| IBIS file generated by GenIBIS323.exe Version 3.23
|   TDA2x
[IBIS ver]   5.0
[File name]   TDA2x.ibs
[File Rev]   1.3.4
[Date]   Mon Apr 15, 2014, 10:23:51
[Source]   Data created at Texas Instruments
[Notes]   TDA2x 23mm IBIS Model Revision History
   TDA2x Version 1.3.4, June 9th, 2014
   - Created TDA2x version from parent device
   - Does not apply to TDA2Ex device
   Version 1.3.4, April 15, 2014
   - Added new 1-2-1 package RLC data
   Version 1.3.3, September 20, 2013
   - Updated the following models to more accurately
   represent the slew and delay characteristics.
   * Models include:
   > bc1833dv40dcpbfbhhvrxp1811_sscev
   > bc1833dv40dcpbfbp1811_ssceh
   > bc1833dv40dcpbfbp1811_sscev
   > bi2c1833dvfzp18_sscev
   > iq1833dvtckpbfbp18ll_sscev
   * Peripherals that use the corresponding IO buffers
   include:
   > GPMC
   > VIN/VOUT
   > MDIO
   > RGMII
   > UART
   > McASP
   > GPIO
   > MMC
   > SPI
   > DCAN
   > I2C
   > USB (AB10,AC10)
   > Debug
   > System and Misc Signals
   Version 1.3.2, August 14, 2013
   - Updated DDR models to address the minimum supply
   voltage and the discontinuities in the vertical
   single ended models.
   Version 1.3.1, August 5, 2013
   - Updated DDR2 (1.8V) models; regenerated at 400 MHz
   Version 1.3.0, June 14, 2013
   - Added I2C models
   - Added MLB models
   - Added DDR Clock pins as differential
   Version 1.2.0, May 23, 2013
   - Added DDR2 (1.8V) models
   - Added DDR DQS pins as differential
   Version 1.1.1, April 8, 2013
   - Modifications, Additions, Deletions
   * Changed name of file to be package specific
   * Updated the following source IO models:
   > DDR_SEIOPB_V
   > DDR_SEIOPB_H
   > DDR_DIFFIOPB_H
   * Replaced the following source IO models:
   > GANGARX_HMAV10GS80 with GANGARX
   > SHANTANUTX_HMAV10GS80 with
   USB3_PCIEGEN1_PCIEGEN2_TX / SATATX
   * Added the following source IO models:
   > ACSPCIE_RX
   > IHHV1833DVHYP1811_SSCEV
   > BC1833DV40DCPBFBHHVRXP1811_SSCEV
   > IQ1833DVTCKPBFBP18LL_SSCEV
   * Changed source IO buffer model to existing model
   > For some pins, the following two models were
   interchanged: BC1833DV40DCPBFBP1811_SSCEH,
   BC1833DV40DCPBFBP1811_SSCEV
   * Updated the RLC data for all pins
   * Changed the supported DDR voltage from 1.2V/1.5V
   to 1.35/1.5V for DDR3 usage
   Version 1.0, January 16, 2013
   - Initial Release
   Note 1) Checked by IBISCHK5.
   Note 2) Interfaces Included in this IBIS Model
   - DDR1,2
   - GPIO6
   - GPMC
   - VIP1
   - VIP2
   - DSS
   - HDMI1
   - RGMII
   - UART3
   - USB1,2
   - PCIE
   - XREFCLK
   - McASP1,2,3,4,5
   - MMC1,3
   - SPI1,2
   - DCAN
   - UART1,2,3
   - SATA1
   - I2C1
   - I2C2
   - MLB
[Disclaimer] Please be aware that in the absence of a written agreement,
   Texas Instruments (TI) assumes no liability for: 1) the
   accuracy of the IBIS models provided to your company, 2) the
   proper functioning of these IBIS models in your design or for
   any resulting applications, or, 3) infringement of patents,
   copyrights, or intellectual property rights resulting from
   your use of these IBIS models. TI provides IBIS models as a
   service to our customers and therefore reserves the right to
   limit distribution of the IBIS models.
[Copyright]   Property of Texas Instruments Incorporated. Unauthorised
   reproduction and/or distribution is strictly prohibited. This
   product is protected under copyright law and trade secret law
   as an unpublished work. Created 2013,(C) Copyright 2013,
   Texas Instruments Incorporated., All Rights Reserved. These
   commodities are under the U.S. Government distribution license
   control.As such,they are not to be re-exported without the
   prior approval of the U.S. Department of Commerce.
|   Component TDA2x
[Component]   TDA2x
[Manufacturer]   Texas Instruments.
| Source IO level model revisions
|Model   Revision   Date
|ILVDS18HY_SSCEH   1.0   Apr 04, 2013
|BMLBLVDS18_SSCEH   1.0   Jun 13, 2013
|BC1833DV40DCPBFBP1811_SSCEH   2.0   Sep 11, 2013
|DDR_SEIOPB_H   2.4   14 Aug 2013
|GANGARX   1   Sep 04, 2012
|SDIO1833PB_H   1.0   Sep 21, 2011
|IQ1833DVTCKPBFBP18LL_SSCEV   2.0   Sep 11, 2013
|USB3_PCIEGEN1_PCIEGEN2_TX   1.0   Nov 07, 2012
|ACSPCIE_RX   0.5   May 16, 2012
|BI2C1833DVFZP18_SSCEV   2.0   Sep 11, 2013
|IHHV1833DVHYP1811_SSCEV   1.0   Dec 24, 2012
|DDR_SEIOPB_V   2.4   14 Aug 2013
|DDR_DIFFIOPB_H   2.4   14 Aug 2013
|HDMITXPHY   0.8   Jul 12, 2011
|DDR_DIFFIOPB_V   2.4   14 Aug 2013
|USB2PHYCORE_HMAV10GS80   0.8   July 13, 2011
|BC1833DV40DCPBFBP1811_SSCEV   2.0   Sep 11, 2013
|SATATX   1.0   Nov 07, 2012
|BC1833DV40DCPBFBHHVRXP1811_SSCEV   2.0   Sep 11, 2013
[Package]
|   typ   min   max
R_pkg   0.410630813888888   0.0487026   0.806879
L_pkg   5.77142293162393E-009 8.65672E-10   1.23044E-08
C_pkg   7.4889892948718E-013 2.85269E-13   1.26574E-12
[Pin]   signal_name   model_name   R_pin   L_pin   C_pin
Y10   ATESTV   NC
G19   DCAN1_RX   Selector_10  0.142301   1.81835E-09 4.38728E-13
G20   DCAN1_TX   Selector_10  0.137913   1.91785E-09 4.43391E-13
AA25   DDR1_D30   Selector_9   0.488374   6.55624E-09 9.83881E-13
AC26   DDR1_DQM2   Selector_23  0.571621   7.36463E-09 7.5871E-13
AA27   DDR1_DQM3   Selector_23  0.505641   7.39922E-09 8.05209E-13
AH22   DDR1_A5   Selector_14  0.489767   6.96396E-09 8.56083E-13
Y27   DDR1_DQSN3   Selector_22  0.468375   7.13463E-09 6.18565E-13
AA26   DDR1_D29   Selector_9   0.504051   6.68279E-09 8.96047E-13
Y20   DDR1_D23   Selector_9   0.455055   4.62626E-09 9.31601E-13
AF25   DDR1_D0   Selector_9   0.547194   7.82073E-09 8.17645E-13
AD27   DDR1_DQS2   Selector_2   0.511052   7.93612E-09 6.63607E-13
V20   DDR1_D16   Selector_9   0.496658   4.60207E-09 6.66551E-13
AE28   DDR1_DQSN1   Selector_22  0.52608   8.75962E-09 6.7652E-13
W22   DDR1_ECC_D0   Selector_9   0.391173   4.73415E-09 8.7308E-13
W20   DDR1_D17   Selector_9   0.476985   4.28121E-09 8.48532E-13
Y23   DDR1_D26   Selector_9   0.479951   5.39702E-09 8.38804E-13
AD20   DDR1_A0   Selector_14  0.491074   4.69941E-09 7.61683E-13
AD22   DDR1_A11   Selector_14  0.464556   5.06886E-09 7.34666E-13
AD18   DDR1_A15   Selector_14  0.477384   4.97278E-09 7.25895E-13
AH25   DDR1_DQS0   Selector_2   0.491307   7.94468E-09 6.51776E-13
AF28   DDR1_D11   Selector_9   0.563042   8.80825E-09 9.29844E-13
AH21   DDR1_WEN   Selector_14  0.490909   6.72126E-09 7.52517E-13
AC18   DDR1_CASN   Selector_14  0.479809   4.10908E-09 9.02863E-13
Y25   DDR1_ECC_D4   Selector_9   0.433519   6.03553E-09 8.75322E-13
AF23   DDR1_D6   Selector_9   0.525055   6.82231E-09 9.6887E-13
AC19   DDR1_A1   Selector_14  0.465932   4.58919E-09 8.99261E-13
AE24   DDR1_D5   Selector_9   0.567056   6.70164E-09 8.95563E-13
AF21   DDR1_A4   Selector_14  0.465648   5.66338E-09 8.01622E-13
AE21   DDR1_A7   Selector_14  0.4759   5.50088E-09 7.72657E-13
AC27   DDR1_D20   Selector_9   0.548177   7.71401E-09 9.67757E-13
AA24   DDR1_D27   Selector_9   0.485891   5.99486E-09 1.02065E-12
V28   DDR1_DQSN_ECC   Selector_22  0.428445   6.8489E-09 5.83984E-13
AH23   DDR1_CSN0   Selector_14  0.485959   7.33449E-09 8.46496E-13
V25   DDR1_ECC_D6   Selector_9   0.442687   5.42329E-09 8.91358E-13
AE26   DDR1_D12   Selector_9   0.564674   7.86732E-09 1.01558E-12
W19   DDR1_ECC_D2   Selector_9   0.305263   4.60654E-09 4.91779E-13
AF27   DDR1_D9   Selector_9   0.565294   8.17506E-09 1.03913E-12
V24   DDR1_ECC_D5   Selector_9   0.433492   5.15658E-09 1.03737E-12
AD23   DDR1_DQM0   Selector_23  0.535358   5.90176E-09 7.25313E-13
AC21   DDR1_A12   Selector_14  0.444582   4.2461E-09 6.71249E-13
Y18   DDR1_VREF0   NC
AF22   DDR1_A8   Selector_14  0.482908   5.98594E-09 8.51919E-13
V23   DDR1_ECC_D1   Selector_9   0.410952   4.86996E-09 8.7205E-13
Y28   DDR1_DQS3   Selector_2   0.469432   7.46481E-09 6.15791E-13
AF20   DDR1_RASN   Selector_14  0.492836   6.17494E-09 7.29374E-13
AG24   DDR1_CK   Selector_7   0.463144   7.46419E-09 6.60615E-13
AD28   DDR1_DQSN2   Selector_22  0.510404   8.32224E-09 6.74162E-13
AB18   DDR1_BA2   Selector_14  0.476485   3.73249E-09 7.57707E-13
AC25   DDR1_D13   Selector_9   0.561034   6.53819E-09 9.74056E-13
AH26   DDR1_D3   Selector_9   0.563544   8.67391E-09 9.23805E-13
AG23   DDR1_A6   Selector_14  0.477168   6.94389E-09 7.82961E-13
AF24   DDR1_D4   Selector_9   0.567364   7.24396E-09 9.65163E-13
AA28   DDR1_D31   Selector_9   0.505301   7.57104E-09 8.85626E-13
AB19   DDR1_A3   Selector_14  0.458874   3.63375E-09 7.35145E-13
Y24   DDR1_D28   Selector_9   0.486596   5.86172E-09 1.08233E-12
V27   DDR1_DQS_ECC   Selector_2   0.422662   6.40168E-09 6.29942E-13
AA23   DDR1_D24   Selector_9   0.460929   6.1893E-09 9.79318E-13
AF18   DDR1_A13   Selector_14  0.429673   5.58028E-09 7.25804E-13
AC23   DDR1_D8   Selector_9   0.538858   6.26131E-09 7.73819E-13
AC28   DDR1_D19   Selector_9   0.544104   8.03812E-09 9.71096E-13
AE23   DDR1_D7   Selector_9   0.543229   6.3764E-09 9.88105E-13
AE18   DDR1_BA1   Selector_14  0.448614   5.33588E-09 8.03247E-13
AB23   DDR1_DQM1   Selector_23  0.53767   6.04637E-09 9.46043E-13
Y19   DDR1_D21   Selector_9   0.448452   4.88152E-09 9.80373E-13
AG26   DDR1_D2   Selector_9   0.566242   8.35538E-09 9.98633E-13
AH24   DDR1_NCK   Selector_18  0.463978   7.70005E-09 6.37576E-13
V26   DDR1_DQM_ECC   Selector_23  0.461108   6.09944E-09 7.12956E-13
AE17   DDR1_A14   Selector_14  0.393257   4.55887E-09 6.9875E-13
AG25   DDR1_DQSN0   Selector_22  0.488286   7.6544E-09 6.85193E-13
AE20   DDR1_ODT0   Selector_14  0.493335   5.59178E-09 8.74184E-13
Y22   DDR1_D25   Selector_9   0.455152   5.4378E-09 8.79622E-13
AC24   DDR1_D14   Selector_9   0.562772   6.40383E-09 9.77754E-13
AC20   DDR1_A2   Selector_14  0.474437   4.33433E-09 8.21491E-13
AE22   DDR1_A9   Selector_14  0.451572   5.54208E-09 7.5977E-13
AD25   DDR1_D15   Selector_9   0.563905   7.18622E-09 8.33158E-13
AB27   DDR1_D22   Selector_9   0.548017   7.16469E-09 9.34631E-13
AF17   DDR1_BA0   Selector_14  0.363148   5.09595E-09 7.8349E-13
W23   DDR1_ECC_D3   Selector_9   0.411229   5.50469E-09 8.04349E-13
AB28   DDR1_D18   Selector_9   0.548364   7.9815E-09 8.83095E-13
AF26   DDR1_D1   Selector_9   0.564992   7.96636E-09 8.38444E-13
Y26   DDR1_ECC_D7   Selector_9   0.437804   6.33869E-09 8.243E-13
AG22   DDR1_CKE   Selector_14  0.488524   6.8453E-09 8.89617E-13
AE27   DDR1_DQS1   Selector_2   0.527341   8.41091E-09 7.07295E-13
AD21   DDR1_A10   Selector_14  0.450742   4.90139E-09 7.69093E-13
AG21   DDR1_RST   Selector_14  0.465812   6.64602E-09 6.81961E-13
AG27   DDR1_D10   Selector_9   0.563089   8.64448E-09 9.80341E-13
P25   DDR2_A6   Selector_23  0.453003   5.94758E-09 9.09075E-13
G28   DDR2_DQS0   Selector_2   0.461291   7.57794E-09 6.16914E-13
T23   DDR2_RASN   Selector_23  0.412552   5.07283E-09 9.11349E-13
M25   DDR2_D30   Selector_9   0.429649   4.93162E-09 8.66061E-13
M24   DDR2_D29   Selector_9   0.425194   4.32737E-09 8.16752E-13
R27   DDR2_A3   Selector_23  0.474573   6.03892E-09 8.14153E-13
R25   DDR2_A0   Selector_23  0.480037   5.494E-09  1.03762E-12
H28   DDR2_DQSN1   Selector_22  0.416577   6.83933E-09 5.59439E-13
J24   DDR2_D15   Selector_9   0.445443   4.53076E-09 7.05822E-13
G24   DDR2_DQM1   Selector_23  0.413019   5.05315E-09 9.52893E-13
P27   DDR2_A8   Selector_23  0.478091   6.65855E-09 7.30202E-13
L25   DDR2_D26   Selector_9   0.419384   4.9549E-09 6.50443E-13
F26   DDR2_D4   Selector_9   0.478471   5.90808E-09 8.82784E-13
N23   DDR2_A10   Selector_23  0.424246   5.70493E-09 8.87666E-13
P23   DDR2_A4   Selector_23  0.435404   5.35545E-09 1.03205E-12
H27   DDR2_DQS1   Selector_2   0.41834   6.40587E-09 5.8892E-13
U23   DDR2_BA0   Selector_23  0.429682   5.52565E-09 9.25158E-13
H25   DDR2_D9   Selector_9   0.444286   4.73335E-09 7.78562E-13
K28   DDR2_DQSN2   Selector_22  0.388299   6.17591E-09 5.59537E-13
T22   DDR2_A13   Selector_23  0.435755   4.62863E-09 8.39607E-13
U24   DDR2_CKE   Selector_23  0.417375   6.15441E-09 1.08206E-12
E28   DDR2_D7   Selector_9   0.420185   6.68015E-09 9.52895E-13
J26   DDR2_D14   Selector_9   0.444455   5.43806E-09 8.14335E-13
K22   DDR2_D22   Selector_9   0.407858   3.17351E-09 7.19244E-13
F27   DDR2_D5   Selector_9   0.47131   6.27857E-09 8.77333E-13
N22   DDR2_VREF0   NC
R24   DDR2_RST   Selector_23  0.459467   4.75459E-09 6.10277E-13
N27   DDR2_A9   Selector_23  0.500555   6.42607E-09 8.0858E-13
H24   DDR2_D10   Selector_9   0.444695   4.26735E-09 6.84693E-13
E26   DDR2_D0   Selector_9   0.430381   6.16167E-09 9.3642E-13
G27   DDR2_DQSN0   Selector_22  0.458967   7.12203E-09 6.88688E-13
L26   DDR2_D25   Selector_9   0.434294   5.28274E-09 7.6646E-13
R23   DDR2_ODT0   Selector_23  0.454898   4.84341E-09 9.81403E-13
L23   DDR2_D19   Selector_9   0.405574   3.83659E-09 6.59391E-13
N28   DDR2_A12   Selector_23  0.486579   6.7043E-09 6.97861E-13
H23   DDR2_D8   Selector_9   0.450297   3.89798E-09 5.15707E-13
P26   DDR2_A11   Selector_23  0.27554   5.36883E-09 8.32604E-13
M22   DDR2_DQM3   Selector_23  0.433598   3.74065E-09 6.35021E-13
P24   DDR2_CSN0   Selector_23  0.443812   5.65757E-09 1.04452E-12
U25   DDR2_WEN   Selector_23  0.465624   5.85963E-09 8.43561E-13
K21   DDR2_D18   Selector_9   0.379168   3.3037E-09 6.88322E-13
K23   DDR2_DQM2   Selector_23  0.406601   3.77847E-09 6.3791E-13
J25   DDR2_D13   Selector_9   0.444619   4.87823E-09 7.98274E-13
M23   DDR2_D28   Selector_9   0.427683   3.80719E-09 6.64654E-13
G26   DDR2_D12   Selector_9   0.443789   5.60773E-09 8.27383E-13
U26   DDR2_BA2   Selector_23  0.479623   5.80667E-09 9.01941E-13
L27   DDR2_D24   Selector_9   0.434949   6.03771E-09 8.29766E-13
M27   DDR2_DQSN3   Selector_22  0.404049   6.195E-09  5.77957E-13
P22   DDR2_A5   Selector_23  0.429797   5.34435E-09 9.09059E-13
J23   DDR2_D21   Selector_9   0.35896   4.27659E-09 7.56671E-13
E27   DDR2_D6   Selector_9   0.424828   6.27032E-09 8.80003E-13
M26   DDR2_D31   Selector_9   0.428812   5.21643E-09 7.91056E-13
K20   DDR2_D17   Selector_9   0.363681   2.97052E-09 7.84333E-13
R28   DDR2_A2   Selector_23  0.440338   6.66525E-09 8.68351E-13
M28   DDR2_DQS3   Selector_2   0.403534   6.65019E-09 5.74802E-13
F25   DDR2_D2   Selector_9   0.475806   5.54542E-09 9.76788E-13
L24   DDR2_D20   Selector_9   0.405479   4.09588E-09 6.63414E-13
F28   DDR2_DQM0   Selector_23  0.496294   7.81995E-09 5.88209E-13
H26   DDR2_D11   Selector_9   0.445756   5.128E-09  8.01138E-13
K27   DDR2_DQS2   Selector_2   0.389027   5.94231E-09 5.4361E-13
R22   DDR2_A14   Selector_23  0.431613   4.10396E-09 7.31404E-13
G25   DDR2_D1   Selector_9   0.491438   5.25161E-09 6.80725E-13
U28   DDR2_CASN   Selector_23  0.479485   6.88158E-09 8.56654E-13
L28   DDR2_D27   Selector_9   0.431477   6.08946E-09 7.63716E-13
T27   DDR2_NCK   Selector_19  0.451957   6.99093E-09 6.55098E-13
U27   DDR2_BA1   Selector_23  0.48795   6.26323E-09 8.69074E-13
R26   DDR2_A1   Selector_23  0.445263   5.56403E-09 1.06848E-12
J20   DDR2_D23   Selector_9   0.351626   3.25197E-09 7.55244E-13
F24   DDR2_D3   Selector_9   0.475631   5.2045E-09 8.98858E-13
T28   DDR2_CK   Selector_20  0.45108   7.27277E-09 6.2314E-13
L22   DDR2_D16   Selector_9   0.402625   3.21383E-09 6.02036E-13
N20   DDR2_A7   Selector_23  0.432107   3.79928E-09 8.42539E-13
U22   DDR2_A15   Selector_23  0.407669   5.35849E-09 8.89981E-13
G21   EMU0   Selector_10  0.183887   2.70625E-09 5.53086E-13
D24   EMU1   Selector_10  0.571856   8.40046E-09 1.04504E-12
F21   GPIO6_16   Selector_10  0.225689   3.20669E-09 5.5591E-13
E21   GPIO6_14   Selector_10  0.303084   4.38462E-09 5.03666E-13
AC5   GPIO6_10   Selector_5   0.474075   6.7728E-09 8.64123E-13
AB4   GPIO6_11   Selector_5   0.421245   6.01837E-09 7.04268E-13
F20   GPIO6_15   Selector_10  0.212065   2.77626E-09 4.91169E-13
P3   GPMC_A17   Selector_5   0.371938   5.45505E-09 7.36827E-13
R6   GPMC_A0   Selector_5   0.217732   2.94649E-09 5.55936E-13
J4   GPMC_A24   Selector_5   0.247695   3.62428E-09 5.05395E-13
J3   GPMC_AD13   Selector_5   0.315242   4.72363E-09 6.92293E-13
L1   GPMC_AD8   Selector_5   0.449743   6.93734E-09 7.28573E-13
P5   GPMC_A7   Selector_5   0.246699   3.17065E-09 5.81908E-13
P6   GPMC_A4   Selector_5   0.17379   2.40117E-09 5.00132E-13
P1   GPMC_CS3   Selector_5   0.486377   7.23655E-09 7.86426E-13
M7   GPMC_A20   Selector_5   0.237756   4.28796E-09 8.09544E-13
L5   GPMC_AD2   Selector_5   0.21652   3.006E-09  5.05478E-13
R3   GPMC_A13   Selector_5   0.417385   5.8408E-09 8.1052E-13
L4   GPMC_AD5   Selector_5   0.237065   3.57808E-09 5.1762E-13
H5   GPMC_A27   Selector_5   0.220691   3.08692E-09 4.66919E-13
P4   GPMC_A12   Selector_5   0.270486   3.84668E-09 6.33659E-13
J1   GPMC_AD10   Selector_5   0.461393   6.84793E-09 7.51707E-13
M1   GPMC_AD3   Selector_5   0.431467   6.64752E-09 6.5277E-13
T9   GPMC_A1   Selector_5   0.297577   4.20392E-09 7.47103E-13
H2   GPMC_AD14   Selector_5   0.424887   6.22548E-09 7.87734E-13
M6   GPMC_AD0   Selector_5   0.0623967  1.73897E-09 4.65864E-13
N6   GPMC_BEN0   Selector_5   0.181144   2.4119E-09 5.23354E-13
M2   GPMC_AD1   Selector_5   0.36614   5.551E-09  6.95395E-13
R2   GPMC_A18   Selector_5   0.426261   6.45202E-09 8.30275E-13
J6   GPMC_A25   Selector_5   0.161418   2.31366E-09 4.44825E-13
R4   GPMC_A9   Selector_5   0.364075   4.69363E-09 6.6057E-13
N9   GPMC_A10   Selector_5   0.0704516  1.39445E-09 3.71414E-13
L6   GPMC_AD4   Selector_5   0.0628788  1.65793E-09 4.75715E-13
R5   GPMC_A6   Selector_5   0.314166   4.15121E-09 6.70616E-13
M4   GPMC_BEN1   Selector_5   0.284796   3.91097E-09 5.91591E-13
H1   GPMC_AD12   Selector_5   0.49008   7.25447E-09 7.7463E-13
T6   GPMC_A2   Selector_5   0.310609   4.31386E-09 6.68677E-13
J2   GPMC_AD11   Selector_5   0.37862   5.63845E-09 7.86007E-13
T1   GPMC_CS0   Selector_5   0.547747   8.08251E-09 8.63303E-13
H6   GPMC_CS1   Selector_5   0.15283   2.16164E-09 3.54794E-13
H3   GPMC_AD15   Selector_5   0.366945   5.27839E-09 6.29529E-13
T2   GPMC_A14   Selector_5   0.45378   6.55015E-09 8.93429E-13
U2   GPMC_A15   Selector_5   0.539544   7.78702E-09 9.79267E-13
N1   GPMC_ADVN_ALE   Selector_5   0.473783   6.96964E-09 7.42842E-13
N2   GPMC_WAIT0   Selector_5   0.382117   5.7663E-09 7.56475E-13
J5   GPMC_A21   Selector_5   0.188381   2.77218E-09 4.57131E-13
P7   GPMC_CLK   Selector_5   0.0817759  1.29823E-09 4.9009E-13
R9   GPMC_A5   Selector_5   0.251842   3.75325E-09 6.67436E-13
K7   GPMC_A19   Selector_5   0.111553   1.59599E-09 4.21047E-13
U1   GPMC_A16   Selector_5   0.539046   7.94879E-09 8.44175E-13
N7   GPMC_A8   Selector_5   0.182345   2.10979E-09 5.97325E-13
M3   GPMC_WEN   Selector_5   0.345682   4.91728E-09 6.73703E-13
J7   GPMC_A23   Selector_5   0.10285   1.48507E-09 3.77069E-13
T7   GPMC_A3   Selector_5   0.212634   3.28461E-09 7.98296E-13
P2   GPMC_CS2   Selector_5   0.397616   5.96876E-09 7.88128E-13
M5   GPMC_OEN_REN   Selector_5   0.199781   2.88885E-09 5.41255E-13
P9   GPMC_A11   Selector_5   0.120642   2.00577E-09 5.14429E-13
L2   GPMC_AD7   Selector_5   0.359214   5.58E-09   6.93076E-13
L3   GPMC_AD6   Selector_5   0.325981   4.87955E-09 6.17128E-13
H4   GPMC_A26   Selector_5   0.252297   3.65141E-09 5.21147E-13
K2   GPMC_AD9   Selector_5   0.351971   5.59305E-09 6.4468E-13
K6   GPMC_A22   Selector_5   0.200506   2.50226E-09 4.82556E-13
AH16   HDMI1_CLOCKY   Model_560   0.522079   6.86158E-09 5.59959E-13
AH17   HDMI1_DATA0Y   Model_560   0.54149   6.98311E-09 5.71255E-13
AH19   HDMI1_DATA2Y   Model_560   0.540501   7.19948E-09 5.3239E-13
AG16   HDMI1_CLOCKX   Model_559   0.519718   6.47654E-09 5.30151E-13
AH18   HDMI1_DATA1Y   Model_560   0.526848   7.01394E-09 5.91894E-13
AG18   HDMI1_DATA1X   Model_559   0.513665   6.3596E-09 6.08132E-13
AG19   HDMI1_DATA2X   Model_559   0.540457   6.6137E-09 5.66E-13
AG17   HDMI1_DATA0X   Model_559   0.537899   6.51607E-09 5.86014E-13
C20   I2C1_SCL   Selector_4   0.391047   5.4679E-09 7.3579E-13
F17   I2C2_SCL   Selector_4   0.158122   2.18035E-09 5.01077E-13
C21   I2C1_SDA   Selector_4   0.395798   5.82709E-09 8.22531E-13
C25   I2C2_SDA   Selector_4   0.64304   9.74271E-09 8.75737E-13
AH15   LJCB_CLKN   Model_228   0.403117   6.62067E-09 5.54035E-13
AG15   LJCB_CLKP   Model_228   0.402119   6.35043E-09 5.88998E-13
E12   MCASP1_AXR4   Selector_10  0.228305   3.05529E-09 5.26292E-13
B14   MCASP1_ACLKR   Selector_10  0.333237   4.81969E-09 7.15725E-13
G13   MCASP1_AXR2   Selector_10  0.114295   1.47199E-09 4.72026E-13
A11   MCASP1_AXR9   Selector_10  0.464424   7.04465E-09 6.57801E-13
G12   MCASP1_AXR0   Selector_10  0.073142   1.12741E-09 4.05063E-13
D14   MCASP1_FSX   Selector_10  0.211293   3.11931E-09 5.35981E-13
G14   MCASP1_AXR14   Selector_10  0.0863827  1.28604E-09 3.83913E-13
A13   MCASP1_AXR13   Selector_10  0.42527   6.56476E-09 5.94071E-13
F13   MCASP1_AXR5   Selector_10  0.174435   2.31626E-09 4.87766E-13
J14   MCASP1_FSR   Selector_10  0.0840519  1.73626E-09 4.10338E-13
F12   MCASP1_AXR1   Selector_10  0.198543   2.73603E-09 4.43901E-13
D12   MCASP1_AXR7   Selector_10  0.306932   4.14247E-09 6.01975E-13
B13   MCASP1_AXR10   Selector_10  0.341508   5.24253E-09 5.92989E-13
F14   MCASP1_AXR15   Selector_10  0.169375   2.29132E-09 5.17262E-13
E14   MCASP1_AXR12   Selector_10  0.156942   2.36734E-09 4.7303E-13
C12   MCASP1_AXR6   Selector_10  0.301133   4.39688E-09 6.02341E-13
B12   MCASP1_AXR8   Selector_10  0.356083   5.48275E-09 6.84897E-13
A12   MCASP1_AXR11   Selector_10  0.453413   6.77542E-09 6.85085E-13
J11   MCASP1_AXR3   Selector_10  0.119381   2.55805E-09 4.46864E-13
C14   MCASP1_ACLKX   Selector_10  0.300587   4.21014E-09 6.59559E-13
A16   MCASP2_AXR3   Selector_10  0.457713   6.69343E-09 7.33522E-13
A19   MCASP2_ACLKX   Selector_10  0.494883   7.09629E-09 9.14831E-13
D15   MCASP2_AXR4   Selector_10  0.223435   3.32269E-09 5.09043E-13
E15   MCASP2_ACLKR   Selector_10  0.167616   2.44562E-09 5.26745E-13
B17   MCASP2_AXR6   Selector_10  0.386872   5.64767E-09 8.13023E-13
B15   MCASP2_AXR0   Selector_10  0.339198   4.95506E-09 7.08087E-13
A18   MCASP2_FSX   Selector_10  0.491953   7.1144E-09 8.6026E-13
A17   MCASP2_AXR7   Selector_10  0.478281   6.88289E-09 7.65246E-13
B16   MCASP2_AXR5   Selector_10  0.39105   5.71425E-09 6.59015E-13
C15   MCASP2_AXR2   Selector_10  0.286526   4.21946E-09 6.25958E-13
A20   MCASP2_FSR   Selector_10  0.587114   8.31311E-09 9.65058E-13
A15   MCASP2_AXR1   Selector_10  0.427106   6.14083E-09 7.35618E-13
F15   MCASP3_FSX   Selector_10  0.133705   1.94098E-09 4.44576E-13
C17   MCASP3_AXR1   Selector_10  0.337685   4.93957E-09 7.35535E-13
B18   MCASP3_ACLKX   Selector_10  0.401825   5.92738E-09 7.6619E-13
B19   MCASP3_AXR0   Selector_10  0.442813   6.49939E-09 8.16848E-13
A21   MCASP4_FSX   Selector_10  0.565932   8.20173E-09 7.75959E-13
D17   MCASP4_AXR1   Selector_10  0.285355   4.15641E-09 6.26235E-13
C18   MCASP4_ACLKX   Selector_10  0.388397   5.6512E-09 7.66903E-13
G16   MCASP4_AXR0   Selector_10  0.0487026  8.65672E-10 3.48812E-13
AB9   MCASP5_FSX   Selector_5   0.325941   5.45548E-09 8.14938E-13
AB3   MCASP5_AXR0   Selector_5   0.492311   7.09349E-09 8.54119E-13
AA3   MCASP5_ACLKX   Selector_5   0.511911   7.19161E-09 9.20097E-13
AA4   MCASP5_AXR1   Selector_5   0.454434   6.37098E-09 9.524E-13
U4   MDIO_D   Selector_5   0.341124   4.78757E-09 5.9896E-13
V1   MDIO_MCLK   Selector_5   0.51993   7.51745E-09 7.08846E-13
AA1   MLBP_DAT_P   Selector_24  0.55177   8.30718E-09 8.24094E-13
AB2   MLBP_CLK_N   Selector_16  0.577275   8.5551E-09 8.28238E-13
AC2   MLBP_SIG_N   Selector_24  0.608531   9.0761E-09 9.41859E-13
AA2   MLBP_DAT_N   Selector_24  0.538816   7.88164E-09 8.8769E-13
AB1   MLBP_CLK_P   Selector_16  0.604449   9.05817E-09 8.03775E-13
AC1   MLBP_SIG_P   Selector_24  0.634373   9.59228E-09 9.40549E-13
Y3   MMC1_DAT3   Selector_8   0.4074   6.2443E-09 6.80906E-13
AA6   MMC1_DAT0   Selector_8   0.442363   6.52582E-09 8.08037E-13
W6   MMC1_CLK   Selector_8   0.259651   3.7484E-09 5.40025E-13
Y4   MMC1_DAT1   Selector_8   0.396318   5.84067E-09 7.55107E-13
W7   MMC1_SDCD   Selector_5   0.200559   3.05745E-09 6.08795E-13
Y5   MMC1_BIAS   NC
Y9   MMC1_SDWP   Selector_5   0.265805   4.36306E-09 7.68518E-13
Y6   MMC1_CMD   Selector_8   0.364922   5.24738E-09 7.32387E-13
AA5   MMC1_DAT2   Selector_8   0.428458   6.3354E-09 8.44641E-13
AC4   MMC3_CMD   Selector_5   0.491307   7.06115E-09 9.39975E-13
AB8   MMC3_DAT6   Selector_5   0.329544   5.1917E-09 8.05247E-13
AC9   MMC3_DAT2   Selector_5   0.424225   6.7789E-09 1.07741E-12
AC7   MMC3_DAT0   Selector_5   0.386933   5.80343E-09 8.99199E-13
AC3   MMC3_DAT3   Selector_5   0.504731   7.31407E-09 8.65115E-13
AD4   MMC3_CLK   Selector_5   0.492472   7.29914E-09 9.80419E-13
AD6   MMC3_DAT5   Selector_5   0.463916   6.93237E-09 8.926E-13
AC8   MMC3_DAT4   Selector_5   0.48249   7.22682E-09 1.01836E-12
AB5   MMC3_DAT7   Selector_5   0.358088   5.27735E-09 7.97562E-13
AC6   MMC3_DAT1   Selector_5   0.39954   5.77264E-09 8.56103E-13
D21   NMIN   Selector_17  0.376251   5.33942E-09 6.41426E-13
Y11   ON_OFF   Selector_11  0.317728   5.12671E-09 6.19734E-13
AH14   PCIE_TXP0   Selector_6   0.403925   6.50981E-09 5.33256E-13
AH11   PCIE_RXP1   Model_177   0.410633   6.61242E-09 5.41708E-13
AG13   PCIE_RXN0   Model_177   0.388441   5.73546E-09 5.1117E-13
AH13   PCIE_RXP0   Model_177   0.389797   6.24602E-09 5.23854E-13
AG12   PCIE_TXN1   Selector_3   0.398788   5.94157E-09 5.19476E-13
AH12   PCIE_TXP1   Selector_6   0.400284   6.40489E-09 5.34334E-13
AG11   PCIE_RXN1   Model_177   0.406595   6.29584E-09 5.35129E-13
AG14   PCIE_TXN0   Selector_3   0.40432   6.15993E-09 5.52591E-13
F22   PORZ   Selector_12  0.299593   4.29796E-09 5.52069E-13
E23   RESETN   Selector_17  0.451476   6.52768E-09 6.36246E-13
V6   RGMII0_TXD1   Selector_5   0.293989   4.47188E-09 7.8309E-13
W9   RGMII0_TXC   Selector_5   0.253035   4.6187E-09 8.26194E-13
V5   RGMII0_RXCTL   Selector_5   0.341807   5.0089E-09 7.63357E-13
V4   RGMII0_RXD3   Selector_5   0.403054   5.54234E-09 7.86074E-13
U5   RGMII0_RXC   Selector_5   0.316468   4.36387E-09 7.72102E-13
U6   RGMII0_TXD0   Selector_5   0.277122   3.87086E-09 7.45633E-13
V9   RGMII0_TXCTL   Selector_5   0.160401   3.25025E-09 5.44905E-13
W2   RGMII0_RXD0   Selector_5   0.482079   7.1184E-09 9.41732E-13
V7   RGMII0_TXD3   Selector_5   0.226663   3.65937E-09 8.08541E-13
U7   RGMII0_TXD2   Selector_5   0.200154   2.94081E-09 6.85228E-13
Y2   RGMII0_RXD1   Selector_5   0.53119   7.70741E-09 9.66603E-13
V3   RGMII0_RXD2   Selector_5   0.421387   6.12672E-09 8.6618E-13
U3   RMII_MHZ_50_CLK   Selector_5   0.394228   5.63863E-09 6.4457E-13
F23   RSTOUTN   Selector_13  0.388143   5.72453E-09 5.83927E-13
AE14   RTC_OSC_XI_CLKIN32   NC
AB17   RTC_PORZ   Selector_12  0.107721   2.55139E-09 5.40536E-13
AD14   RTC_OSC_XO   NC
AF14   RTC_ISO   Selector_12  0.277889   4.22207E-09 6.58815E-13
E18   RTCK   Selector_13  0.209175   2.857E-09  5.76997E-13
AH10   SATA1_TXP0   Model_745   0.490457   7.11615E-09 6.07062E-13
AG10   SATA1_TXN0   Model_745   0.49298   7.28764E-09 6.47186E-13
AG9   SATA1_RXP0   Model_177   0.489356   6.94894E-09 6.01955E-13
AH9   SATA1_RXN0   Model_177   0.489423   7.42331E-09 5.94723E-13
B20   SPI1_CS3   Selector_10  0.443086   6.49573E-09 9.00903E-13
B21   SPI1_CS2   Selector_10  0.476328   7.06755E-09 9.21739E-13
A22   SPI1_CS1   Selector_10  0.609717   8.972E-09  9.40571E-13
A24   SPI1_CS0   Selector_10  0.702809   1.04605E-08 1.14186E-12
A25   SPI1_SCLK   Selector_10  0.742529   1.1198E-08 1.26574E-12
B25   SPI1_D0   Selector_10  0.73144   1.10008E-08 1.26458E-12
F16   SPI1_D1   Selector_10  0.13757   2.01841E-09 4.41219E-13
B24   SPI2_CS0   Selector_10  0.644858   9.7543E-09 1.13622E-12
A26   SPI2_SCLK   Selector_10  0.806879   1.23044E-08 1.12444E-12
G17   SPI2_D0   Selector_10  0.105975   1.4804E-09 4.13765E-13
B22   SPI2_D1   Selector_10  0.552633   8.15846E-09 1.0009E-12
E20   TCLK   Selector_15  0.286763   4.08981E-09 5.81714E-13
D23   TDI   Selector_17  0.506015   7.58584E-09 8.378E-13
F19   TDO   Selector_13  0.17133   2.43892E-09 4.13851E-13
F18   TMS   Selector_17  0.149589   2.17908E-09 4.52193E-13
D20   TRSTN   Selector_17  0.324953   4.78518E-09 5.12269E-13
C26   UART1_TXD   Selector_10  0.578406   8.18946E-09 9.69813E-13
C27   UART1_RTSN   Selector_10  0.597567   8.49589E-09 1.07744E-12
B27   UART1_RXD   Selector_10  0.630058   9.05947E-09 1.05367E-12
E25   UART1_CTSN   Selector_10  0.491036   6.78327E-09 9.89268E-13
D27   UART2_CTSN   Selector_10  0.577314   8.22878E-09 9.99064E-13
C28   UART2_RTSN   Selector_10  0.658967   9.39381E-09 1.12806E-12
D28   UART2_RXD   Selector_10  0.612966   9.00395E-09 9.68164E-13
D26   UART2_TXD   Selector_10  0.503252   7.17941E-09 9.2517E-13
Y1   UART3_TXD   Selector_5   0.55597   8.33467E-09 9.02709E-13
V2   UART3_RXD   Selector_5   0.466962   6.77905E-09 7.8047E-13
AC11   USB_TXN0   Selector_3   0.16771   2.41602E-09 4.75415E-13
AF12   USB_RXN0   Model_177   0.291712   4.62869E-09 5.65358E-13
AE12   USB_RXP0   Model_177   0.281243   4.28708E-09 6.36229E-13
AD11   USB_TXP0   Selector_6   0.173562   2.8275E-09 4.57844E-13
AB10   USB1_DRVVBUS   Selector_5   0.140838   2.36502E-09 4.72136E-13
AD12   USB1_DP   Selector_21  0.260716   4.44808E-09 5.35578E-13
AC12   USB1_DM   Selector_1   0.245527   3.94342E-09 5.6847E-13
AC10   USB2_DRVVBUS   Selector_5   0.193741   3.2117E-09 6.94811E-13
AF11   USB2_DM   Selector_1   0.316979   5.0434E-09 5.51736E-13
AE11   USB2_DP   Selector_21  0.290445   4.66401E-09 6.81983E-13
AG5   VIN1A_D11   Selector_5   0.572162   8.78008E-09 1.02212E-12
AF2   VIN1A_D12   Selector_5   0.653639   1.01776E-08 1.12342E-12
AF8   VIN1A_VSYNC0   Selector_5   0.389003   6.11304E-09 7.93225E-13
AD2   VIN1A_D22   Selector_5   0.619331   9.18019E-09 9.29349E-13
AH6   VIN1A_D3   Selector_5   0.547213   8.4106E-09 9.13072E-13
AG7   VIN1A_D2   Selector_5   0.445823   7.0571E-09 8.36427E-13
AE6   VIN1A_D21   Selector_5   0.456591   6.88554E-09 8.87379E-13
AH4   VIN1A_D7   Selector_5   0.639417   9.87339E-09 1.09308E-12
AF6   VIN1A_D13   Selector_5   0.492037   7.55246E-09 9.23194E-13
AE9   VIN1A_HSYNC0   Selector_5   0.340215   5.2259E-09 6.62958E-13
AG4   VIN1A_D8   Selector_5   0.597057   9.24078E-09 1.0824E-12
AE8   VIN1A_D0   Selector_5   0.358322   5.4047E-09 7.13097E-13
AE1   VIN1A_D19   Selector_5   0.701732   1.04881E-08 1.16106E-12
AH5   VIN1A_D5   Selector_5   0.563522   9.01817E-09 1.00621E-12
AF4   VIN1A_D15   Selector_5   0.559425   8.59373E-09 1.03495E-12
AG6   VIN1A_D6   Selector_5   0.512309   7.8416E-09 9.01794E-13
AD3   VIN1A_D23   Selector_5   0.59106   8.51576E-09 1.08642E-12
AG3   VIN1A_D10   Selector_5   0.679451   1.03746E-08 1.18243E-12
AH7   VIN1B_CLK1   Selector_5   0.498469   7.70257E-09 6.58833E-13
AG8   VIN1A_CLK0   Selector_5   0.457532   6.83135E-09 6.6871E-13
AH3   VIN1A_D4   Selector_5   0.668031   1.05012E-08 1.06704E-12
AF1   VIN1A_D16   Selector_5   0.736243   1.13924E-08 1.13948E-12
AE2   VIN1A_D20   Selector_5   0.677012   9.95069E-09 1.16951E-12
AE3   VIN1A_D17   Selector_5   0.582122   8.77862E-09 9.76909E-13
AF9   VIN1A_FLD0   Selector_5   0.406232   6.27381E-09 7.66384E-13
AG2   VIN1A_D9   Selector_5   0.71641   1.09543E-08 1.07208E-12
AE5   VIN1A_D18   Selector_5   0.482048   7.2712E-09 8.61386E-13
AF3   VIN1A_D14   Selector_5   0.633276   9.6697E-09 1.11049E-12
AD9   VIN1A_DE0   Selector_5   0.246028   3.80623E-09 5.09334E-13
AD8   VIN1A_D1   Selector_5   0.24784   3.85994E-09 5.98588E-13
F5   VIN2A_D8   Selector_10  0.293094   4.33384E-09 6.21379E-13
D1   VIN2A_D2   Selector_10  0.53152   8.36283E-09 8.3361E-13
H7   VIN2A_FLD0   Selector_10  0.0992969  1.54536E-09 2.85269E-13
D3   VIN2A_D10   Selector_10  0.482334   7.12756E-09 7.11437E-13
B2   VIN2A_D16   Selector_10  0.670871   9.90886E-09 9.63124E-13
E6   VIN2A_D9   Selector_10  0.289648   4.49359E-09 5.76697E-13
F4   VIN2A_D5   Selector_10  0.342765   5.13597E-09 6.79334E-13
C3   VIN2A_D14   Selector_10  0.564261   8.33582E-09 9.1143E-13
F2   VIN2A_D0   Selector_10  0.434444   6.70369E-09 6.57433E-13
C1   VIN2A_D6   Selector_10  0.603057   9.35372E-09 9.06895E-13
G6   VIN2A_VSYNC0   Selector_10  0.173073   2.60849E-09 4.79283E-13
B3   VIN2A_D20   Selector_10  0.607748   8.92307E-09 1.00772E-12
C2   VIN2A_D13   Selector_10  0.608196   8.93568E-09 9.0051E-13
A3   VIN2A_D19   Selector_10  0.617913   9.30781E-09 1.03327E-12
E1   VIN2A_CLK0   Selector_10  0.492448   7.7286E-09 6.23374E-13
A4   VIN2A_D23   Selector_10  0.608437   8.92405E-09 9.87348E-13
F3   VIN2A_D1   Selector_10  0.397599   5.95487E-09 6.67246E-13
G2   VIN2A_DE0   Selector_10  0.383599   6.00813E-09 6.53405E-13
G1   VIN2A_HSYNC0   Selector_10  0.425177   6.70146E-09 6.20679E-13
E2   VIN2A_D3   Selector_10  0.464346   7.19229E-09 8.33253E-13
F6   VIN2A_D11   Selector_10  0.277678   4.16847E-09 6.13192E-13
D6   VIN2A_D17   Selector_10  0.335356   5.0976E-09 7.27567E-13
B4   VIN2A_D21   Selector_10  0.577374   8.30343E-09 1.04696E-12
E4   VIN2A_D7   Selector_10  0.371435   5.56451E-09 6.82893E-13
C5   VIN2A_D18   Selector_10  0.460076   6.92289E-09 8.854E-13
D5   VIN2A_D12   Selector_10  0.407932   6.12638E-09 7.59215E-13
D2   VIN2A_D4   Selector_10  0.490145   7.64603E-09 8.8904E-13
B5   VIN2A_D22   Selector_10  0.514061   7.53861E-09 7.96783E-13
C4   VIN2A_D15   Selector_10  0.508722   7.52132E-09 8.68113E-13
C6   VOUT1_D13   Selector_10  0.49904   7.27935E-09 8.3304E-13
A7   VOUT1_D18   Selector_10  0.5064   7.71917E-09 8.48373E-13
D11   VOUT1_CLK   Selector_10  0.273445   4.00767E-09 4.59691E-13
E8   VOUT1_D8   Selector_10  0.308615   4.3342E-09 6.40243E-13
E9   VOUT1_D4   Selector_10  0.240997   3.33175E-09 6.17868E-13
D8   VOUT1_D11   Selector_10  0.378176   5.48748E-09 7.58755E-13
G11   VOUT1_D3   Selector_10  0.0749519  1.05964E-09 3.56961E-13
B8   VOUT1_D17   Selector_10  0.411645   6.37086E-09 7.87105E-13
B7   VOUT1_D16   Selector_10  0.48888   7.37144E-09 8.63122E-13
B11   VOUT1_FLD   Selector_10  0.367898   5.56079E-09 6.63263E-13
B10   VOUT1_DE   Selector_10  0.414801   6.2224E-09 7.46377E-13
D7   VOUT1_D10   Selector_10  0.406627   5.99519E-09 7.57925E-13
E7   VOUT1_D7   Selector_10  0.346249   5.1259E-09 7.08654E-13
A10   VOUT1_D23   Selector_10  0.437555   6.76956E-09 7.17642E-13
C11   VOUT1_HSYNC   Selector_10  0.34783   4.97733E-09 6.40453E-13
C8   VOUT1_D14   Selector_10  0.386111   5.74405E-09 7.8139E-13
A9   VOUT1_D21   Selector_10  0.451699   6.97473E-09 7.912E-13
D9   VOUT1_D9   Selector_10  0.295602   4.12439E-09 6.6895E-13
A5   VOUT1_D12   Selector_10  0.577587   8.9407E-09 8.44031E-13
F9   VOUT1_D5   Selector_10  0.231362   3.12245E-09 5.41574E-13
C9   VOUT1_D20   Selector_10  0.371884   5.59635E-09 7.80503E-13
G10   VOUT1_D1   Selector_10  0.138724   1.95045E-09 3.61532E-13
F10   VOUT1_D2   Selector_10  0.14752   2.10623E-09 4.31946E-13
C7   VOUT1_D15   Selector_10  0.447914   6.60457E-09 8.00709E-13
F11   VOUT1_D0   Selector_10  0.0969799  1.56439E-09 4.21602E-13
E11   VOUT1_VSYNC   Selector_10  0.245115   3.4717E-09 4.87406E-13
B9   VOUT1_D22   Selector_10  0.423522   6.45594E-09 8.46955E-13
F8   VOUT1_D6   Selector_10  0.317903   4.36276E-09 6.86393E-13
A8   VOUT1_D19   Selector_10  0.477213   7.41063E-09 8.22924E-13
AD17   WAKEUP0   Selector_12  0.129768   2.65763E-09 7.88928E-13
AC17   WAKEUP1   Selector_12  0.126119   2.51222E-09 6.38717E-13
AB16   WAKEUP2   Selector_12  0.268021   3.97732E-09 8.4237E-13
AC16   WAKEUP3   Selector_12  0.207734   2.82199E-09 7.88651E-13
AC15   XI_OSC1   NC
AE15   XI_OSC0   NC
AD15   XO_OSC0   NC
AC13   XO_OSC1   NC
C23   XREF_CLK3   Selector_10  0.552707   8.07838E-09 7.67259E-13
D18   XREF_CLK0   Selector_10  0.345718   4.8501E-09 6.44294E-13
B26   XREF_CLK2   Selector_10  0.743316   1.13869E-08 9.48433E-13
E17   XREF_CLK1   Selector_10  0.246796   3.38676E-09 5.56428E-13
[Diff Pin] inv_pin vdiff tdelay_typ tdelay_min tdelay_max
|Differential signal data for cell ILVDS18HY_SSCEH
|MLBP_CLK_P   MLBP_CLK_N
AB1   AB2   200m   NA
|Differential signal data for cell BMLBLVDS18_SSCEH
|MLBP_SIG_P   MLBP_SIG_N
AC1   AC2   200m   NA
|MLBP_DAT_P   MLBP_DAT_N
AA1   AA2   200m   NA
|Differential signal data for cell GANGARX
|PCIE_RXP1   PCIE_RXN1
AH11   AG11   100mV  NA
|PCIE_RXP0   PCIE_RXN0
AH13   AG13   100mV  NA
|SATA1_RXP0   SATA1_RXN0
AG9   AH9   100mV  NA
|USB_RXP0   USB_RXN0
AE12   AF12   100mV  NA
|Differential signal data for cell DDR_DIFFIOPB_H
|DDR2_DQS3   DDR2_DQSN3
M28   M27   200m   0
|DDR1_DQS3   DDR1_DQSN3
Y28   Y27   200m   0
|DDR2_DQS2   DDR2_DQSN2
K27   K28   200m   0
|DDR1_DQS_ECC   DDR1_DQSN_ECC
V27   V28   200m   0
|DDR1_DQS1   DDR1_DQSN1
AE27   AE28   200m   0
|DDR1_DQS2   DDR1_DQSN2
AD27   AD28   200m   0
|DDR2_DQS1   DDR2_DQSN1
H27   H28   200m   0
|DDR2_CK   DDR2_NCK
T28   T27   200m   0
|DDR1_DQS0   DDR1_DQSN0
AH25   AG25   200m   0
|DDR2_DQS0   DDR2_DQSN0
G28   G27   200m   0
|Differential signal data for cell USB3_PCIEGEN1_PCIEGEN2_TX
|PCIE_TXP1   PCIE_TXN1
AH12   AG12   200m   0
|USB_TXP0   USB_TXN0
AD11   AC11   200m   0
|PCIE_TXP0   PCIE_TXN0
AH14   AG14   200m   0
|Differential signal data for cell HDMITXPHY
|HDMI1_DATA0X   HDMI1_DATA0Y
AG17   AH17   0.0V   0.0s
|HDMI1_CLOCKX   HDMI1_CLOCKY
AG16   AH16   0.0V   0.0s
|HDMI1_DATA1X   HDMI1_DATA1Y
AG18   AH18   0.0V   0.0s
|HDMI1_DATA2X   HDMI1_DATA2Y
AG19   AH19   0.0V   0.0s
|Differential signal data for cell ACSPCIE_RX
|LJCB_CLKP   LJCB_CLKN
AG15   AH15   150m   NA   NA   NA
|Differential signal data for cell DDR_DIFFIOPB_V
|DDR1_CK   DDR1_NCK
AG24   AH24   200m   0
|Differential signal data for cell USB2PHYCORE_HMAV10GS80
|USB1_DP   USB1_DM
AD12   AC12   200mV 0ns 0ns 0ns
|USB2_DP   USB2_DM
AE11   AF11   200mV 0ns 0ns 0ns
|Differential signal data for cell SATATX
|SATA1_TXP0   SATA1_TXN0
AH10   AG10   200m   0
|   Usage I/O#X###USB2PHYCORE_HMAV10GS80.DM
|   Base model USB2PHYCORE_HMAV10GS80
[Model Selector] Selector_1
Model_723 3-STATE,3.3000V,fsdm_tx
Model_725 3-STATE,3.3000V,lsdm_50pf_tx
Model_727 3-STATE,3.3000V,lsdm_200pf_tx
Model_729 3-STATE,3.3000V,lsdm_400pf_tx
Model_731 3-STATE,3.3000V,lsdm_600pf_tx
Model_732 INPUT,3.3V,fsrx
Model_734 3-STATE,0.8000V,hsdm_tx
Model_735 INPUT,3.3V,hsrx
|   Usage I/O#1.35/1.5/1.8###DDR_DIFFIOPB_H.PADP
|   Base model DDR_DIFFIOPB_H
[Model Selector] Selector_2
Model_478 I/O,1.8V,SR011_DRV48_1P8
Model_479 I/O,1.8V,SR010_DRV48_1P8
Model_480 I/O,1.8V,SR101_DRV48_1P8
Model_481 I/O,1.8V,SR100_DRV48_1P8
Model_482 I/O,1.8V,SR110_DRV48_1P8
Model_483 I/O,1.8V,SR111_DRV48_1P8
Model_484 I/O,1.8V,SR001_DRV48_1P8
Model_485 I/O,1.8V,SR000_DRV48_1P8
Model_486 I/O,1.8V,SR011_DRV40_1P8
Model_487 I/O,1.8V,SR010_DRV40_1P8
Model_488 I/O,1.8V,SR101_DRV40_1P8
Model_489 I/O,1.8V,SR100_DRV40_1P8
Model_490 I/O,1.8V,SR110_DRV40_1P8
Model_491 I/O,1.8V,SR111_DRV40_1P8
Model_492 I/O,1.8V,SR001_DRV40_1P8
Model_493 I/O,1.8V,SR000_DRV40_1P8
Model_494 I/O,1.8V,SR011_DRV34_1P8
Model_495 I/O,1.8V,SR010_DRV34_1P8
Model_496 I/O,1.8V,SR101_DRV34_1P8
Model_497 I/O,1.8V,SR100_DRV34_1P8
Model_498 I/O,1.8V,SR110_DRV34_1P8
Model_499 I/O,1.8V,SR111_DRV34_1P8
Model_500 I/O,1.8V,SR001_DRV34_1P8
Model_501 I/O,1.8V,SR000_DRV34_1P8
Model_502 INPUT,1.5V,DDR3_ODT_80_1P5
Model_503 INPUT,1.5V,DDR3_ODT_60_1P5
Model_504 INPUT,1.5V,DDR3_ODT_120_1P5
Model_505 INPUT,1.35V,DDR3L_ODT_80_1P35
Model_506 INPUT,1.35V,DDR3L_ODT_60_1P35
Model_507 INPUT,1.35V,DDR3L_ODT_120_1P35
Model_508 INPUT,1.8V,DDR2_ODT_120_1P8
Model_509 INPUT,1.8V,DDR2_ODT_80_1P8
Model_510 INPUT,1.8V,DDR2_ODT_60_1P8
Model_511 I/O,1.5V,SR011_DRV40_1P5
Model_512 I/O,1.5V,SR010_DRV40_1P5
Model_513 I/O,1.5V,SR101_DRV40_1P5
Model_514 I/O,1.5V,SR100_DRV40_1P5
Model_515 I/O,1.5V,SR110_DRV40_1P5
Model_516 I/O,1.5V,SR111_DRV40_1P5
Model_517 I/O,1.5V,SR001_DRV40_1P5
Model_518 I/O,1.5V,SR000_DRV40_1P5
Model_519 I/O,1.5V,SR011_DRV34_1P5
Model_520 I/O,1.5V,SR010_DRV34_1P5
Model_521 I/O,1.5V,SR101_DRV34_1P5
Model_522 I/O,1.5V,SR100_DRV34_1P5
Model_523 I/O,1.5V,SR110_DRV34_1P5
Model_524 I/O,1.5V,SR111_DRV34_1P5
Model_525 I/O,1.5V,SR001_DRV34_1P5
Model_526 I/O,1.5V,SR000_DRV34_1P5
Model_527 I/O,1.5V,SR011_DRV48_1P5
Model_528 I/O,1.5V,SR010_DRV48_1P5
Model_529 I/O,1.5V,SR101_DRV48_1P5
Model_530 I/O,1.5V,SR100_DRV48_1P5
Model_531 I/O,1.5V,SR110_DRV48_1P5
Model_532 I/O,1.5V,SR111_DRV48_1P5
Model_533 I/O,1.5V,SR001_DRV48_1P5
Model_534 I/O,1.5V,SR000_DRV48_1P5
Model_535 I/O,1.35V,SR011_DRV40_1P35
Model_536 I/O,1.35V,SR010_DRV40_1P35
Model_537 I/O,1.35V,SR101_DRV40_1P35
Model_538 I/O,1.35V,SR100_DRV40_1P35
Model_539 I/O,1.35V,SR110_DRV40_1P35
Model_540 I/O,1.35V,SR111_DRV40_1P35
Model_541 I/O,1.35V,SR001_DRV40_1P35
Model_542 I/O,1.35V,SR000_DRV40_1P35
Model_543 I/O,1.35V,SR011_DRV34_1P35
Model_544 I/O,1.35V,SR010_DRV34_1P35
Model_545 I/O,1.35V,SR101_DRV34_1P35
Model_546 I/O,1.35V,SR100_DRV34_1P35
Model_547 I/O,1.35V,SR110_DRV34_1P35
Model_548 I/O,1.35V,SR111_DRV34_1P35
Model_549 I/O,1.35V,SR001_DRV34_1P35
Model_550 I/O,1.35V,SR000_DRV34_1P35
Model_551 I/O,1.35V,SR011_DRV48_1P35
Model_552 I/O,1.35V,SR010_DRV48_1P35
Model_553 I/O,1.35V,SR101_DRV48_1P35
Model_554 I/O,1.35V,SR100_DRV48_1P35
Model_555 I/O,1.35V,SR110_DRV48_1P35
Model_556 I/O,1.35V,SR111_DRV48_1P35
Model_557 I/O,1.35V,SR001_DRV48_1P35
Model_558 I/O,1.35V,SR000_DRV48_1P35
|   Usage OUTPUT#X###USB3_PCIEGEN1_PCIEGEN2_TX.TXN
|   Base model USB3_PCIEGEN1_PCIEGEN2_TX
[Model Selector] Selector_3
Model_190 3-STATE,1.1V,USB3_TX_FS_NO_DEEMPHASIS
Model_191 3-STATE,1.1V,USB3_TX_FS_3p5_DEEMPHASIS
Model_192 3-STATE,1.1V,USB3_TX_HS_NO_DEEMPHASIS
Model_193 3-STATE,1.1V,PCIEGEN1_TX_FS_NO_DEEMPHASIS_1p2v
Model_194 3-STATE,1.1V,PCIEGEN1_TX_FS_NO_DEEMPHASIS_0p8v
Model_195 3-STATE,1.1V,PCIEGEN1_TX_FS_NO_DEEMPHASIS_0p6v
Model_196 3-STATE,1.1V,PCIEGEN1_TX_FS_NO_DEEMPHASIS_0p4v
Model_197 3-STATE,1.1V,PCIEGEN1_TX_FS_3p5_DEEMPHASIS_1p2v
Model_198 3-STATE,1.1V,PCIEGEN1_TX_FS_3p5_DEEMPHASIS_0p8v
Model_199 3-STATE,1.1V,PCIEGEN1_TX_FS_3p5_DEEMPHASIS_0p6v
Model_200 3-STATE,1.1V,PCIEGEN1_TX_FS_3p5_DEEMPHASIS_0p4v
Model_201 3-STATE,1.1V,PCIEGEN1_TX_HS_NO_DEEMPHASIS_0p6v
Model_202 3-STATE,1.1V,PCIEGEN1_TX_HS_NO_DEEMPHASIS_0p4v
Model_203 3-STATE,1.1V,PCIEGEN1_TX_HS_NO_DEEMPHASIS_0p3v
Model_204 3-STATE,1.1V,PCIEGEN1_TX_HS_NO_DEEMPHASIS_0p2v
Model_205 3-STATE,1.1V,PCIEGEN2_TX_FS_NO_DEEMPHASIS_1p2v
Model_206 3-STATE,1.1V,PCIEGEN2_TX_FS_NO_DEEMPHASIS_0p8v
Model_207 3-STATE,1.1V,PCIEGEN2_TX_FS_NO_DEEMPHASIS_0p6v
Model_208 3-STATE,1.1V,PCIEGEN2_TX_FS_NO_DEEMPHASIS_0p4v
Model_209 3-STATE,1.1V,PCIEGEN2_TX_FS_3p5_DEEMPHASIS_1p2v
Model_210 3-STATE,1.1V,PCIEGEN2_TX_FS_3p5_DEEMPHASIS_0p8v
Model_211 3-STATE,1.1V,PCIEGEN2_TX_FS_3p5_DEEMPHASIS_0p6v
Model_212 3-STATE,1.1V,PCIEGEN2_TX_FS_3p5_DEEMPHASIS_0p4v
Model_213 3-STATE,1.1V,PCIEGEN2_TX_FS_6p0_DEEMPHASIS_1p2v
Model_214 3-STATE,1.1V,PCIEGEN2_TX_FS_6p0_DEEMPHASIS_0p8v
Model_215 3-STATE,1.1V,PCIEGEN2_TX_FS_6p0_DEEMPHASIS_0p6v
Model_216 3-STATE,1.1V,PCIEGEN2_TX_FS_6p0_DEEMPHASIS_0p4v
Model_217 3-STATE,1.1V,PCIEGEN2_TX_HS_NO_DEEMPHASIS_0p6v
Model_218 3-STATE,1.1V,PCIEGEN2_TX_HS_NO_DEEMPHASIS_0p4v
Model_219 3-STATE,1.1V,PCIEGEN2_TX_HS_NO_DEEMPHASIS_0p3v
Model_220 3-STATE,1.1V,PCIEGEN2_TX_HS_NO_DEEMPHASIS_0p2v
|   Usage I/O#1.8/3.3###BI2C1833DVFZP18_SSCEV.PAD
|   Base model BI2C1833DVFZP18_SSCEV
[Model Selector] Selector_4
Model_229 I/O_OPEN_DRAIN,1.8V,FAST MODE AND STD MODE,IND,10 PERCENT%,FAST_STD_MODE_1.8V_10P_1P8
Model_230 I/O_OPEN_DRAIN,3.3V,FAST MODE AND STD MODE,IND,10 PERCENT%,FAST_STD_MODE_3.3V_10P_3P3
Model_231 I/O_OPEN_DRAIN,1.8V,FAST MODE AND STD MODE,IND,5 PERCENT%,FAST_STD_MODE_1.8V_5P_1P8
Model_232 I/O_OPEN_DRAIN,3.3V,FAST MODE AND STD MODE,IND,5 PERCENT%,FAST_STD_MODE_3.3V_5P_3P3
|   Usage I/O#1.8/3.3###BC1833DV40DCPBFBP1811_SSCEH.PAD
|   Base model BC1833DV40DCPBFBP1811_SSCEH
[Model Selector] Selector_5
Model_168 I/O,1.8V,40D CLASS MODE FAST MODE,IND,10 PERCENT%,BC40D_H_10P_!SC1_1P8
Model_169 I/O,1.8V,40C CLASS MODE SLOW MODE,IND,10 PERCENT%,BC40D_H_10P_SC1_1P8
Model_170 I/O,1.8V,40D CLASS MODE FAST MODE,IND,5 PERCENT%,BC40D_H_5P_!SC1_1P8
Model_171 I/O,1.8V,40C CLASS MODE SLOW MODE,IND,5 PERCENT%,BC40D_H_5P_SC1_1P8
Model_172 I/O,3.3V,40D CLASS MODE FAST MODE,IND,10 PERCENT%,BC40D_H_10P_!SC1_3P3
Model_173 I/O,3.3V,40C CLASS MODE SLOW MODE,IND,10 PERCENT%,BC40D_H_10P_SC1_3P3
Model_174 I/O,3.3V,40D CLASS MODE FAST MODE,IND,5 PERCENT%,BC40D_H_5P_!SC1_3P3
Model_175 I/O,3.3V,40C CLASS MODE SLOW MODE,IND,5 PERCENT%,BC40D_H_5P_SC1_3P3
|   Usage OUTPUT#X###USB3_PCIEGEN1_PCIEGEN2_TX.TXP
|   Base model USB3_PCIEGEN1_PCIEGEN2_TX
[Model Selector] Selector_6
Model_190 3-STATE,1.1V,USB3_TX_FS_NO_DEEMPHASIS
Model_191 3-STATE,1.1V,USB3_TX_FS_3p5_DEEMPHASIS
Model_192 3-STATE,1.1V,USB3_TX_HS_NO_DEEMPHASIS
Model_193 3-STATE,1.1V,PCIEGEN1_TX_FS_NO_DEEMPHASIS_1p2v
Model_194 3-STATE,1.1V,PCIEGEN1_TX_FS_NO_DEEMPHASIS_0p8v
Model_195 3-STATE,1.1V,PCIEGEN1_TX_FS_NO_DEEMPHASIS_0p6v
Model_196 3-STATE,1.1V,PCIEGEN1_TX_FS_NO_DEEMPHASIS_0p4v
Model_197 3-STATE,1.1V,PCIEGEN1_TX_FS_3p5_DEEMPHASIS_1p2v
Model_198 3-STATE,1.1V,PCIEGEN1_TX_FS_3p5_DEEMPHASIS_0p8v
Model_199 3-STATE,1.1V,PCIEGEN1_TX_FS_3p5_DEEMPHASIS_0p6v
Model_200 3-STATE,1.1V,PCIEGEN1_TX_FS_3p5_DEEMPHASIS_0p4v
Model_201 3-STATE,1.1V,PCIEGEN1_TX_HS_NO_DEEMPHASIS_0p6v
Model_202 3-STATE,1.1V,PCIEGEN1_TX_HS_NO_DEEMPHASIS_0p4v
Model_203 3-STATE,1.1V,PCIEGEN1_TX_HS_NO_DEEMPHASIS_0p3v
Model_204 3-STATE,1.1V,PCIEGEN1_TX_HS_NO_DEEMPHASIS_0p2v
Model_205 3-STATE,1.1V,PCIEGEN2_TX_FS_NO_DEEMPHASIS_1p2v
Model_206 3-STATE,1.1V,PCIEGEN2_TX_FS_NO_DEEMPHASIS_0p8v
Model_207 3-STATE,1.1V,PCIEGEN2_TX_FS_NO_DEEMPHASIS_0p6v
Model_208 3-STATE,1.1V,PCIEGEN2_TX_FS_NO_DEEMPHASIS_0p4v
Model_209 3-STATE,1.1V,PCIEGEN2_TX_FS_3p5_DEEMPHASIS_1p2v
Model_210 3-STATE,1.1V,PCIEGEN2_TX_FS_3p5_DEEMPHASIS_0p8v
Model_211 3-STATE,1.1V,PCIEGEN2_TX_FS_3p5_DEEMPHASIS_0p6v
Model_212 3-STATE,1.1V,PCIEGEN2_TX_FS_3p5_DEEMPHASIS_0p4v
Model_213 3-STATE,1.1V,PCIEGEN2_TX_FS_6p0_DEEMPHASIS_1p2v
Model_214 3-STATE,1.1V,PCIEGEN2_TX_FS_6p0_DEEMPHASIS_0p8v
Model_215 3-STATE,1.1V,PCIEGEN2_TX_FS_6p0_DEEMPHASIS_0p6v
Model_216 3-STATE,1.1V,PCIEGEN2_TX_FS_6p0_DEEMPHASIS_0p4v
Model_217 3-STATE,1.1V,PCIEGEN2_TX_HS_NO_DEEMPHASIS_0p6v
Model_218 3-STATE,1.1V,PCIEGEN2_TX_HS_NO_DEEMPHASIS_0p4v
Model_219 3-STATE,1.1V,PCIEGEN2_TX_HS_NO_DEEMPHASIS_0p3v
Model_220 3-STATE,1.1V,PCIEGEN2_TX_HS_NO_DEEMPHASIS_0p2v
|   Usage OUTPUT#1.35/1.5/1.8###DDR_DIFFIOPB_V.PADP
|   Base model DDR_DIFFIOPB_V
[Model Selector] Selector_7
Model_641 I/O,1.8V,SR011_DRV48_1P8
Model_642 I/O,1.8V,SR010_DRV48_1P8
Model_643 I/O,1.8V,SR101_DRV48_1P8
Model_644 I/O,1.8V,SR100_DRV48_1P8
Model_645 I/O,1.8V,SR110_DRV48_1P8
Model_646 I/O,1.8V,SR111_DRV48_1P8
Model_647 I/O,1.8V,SR001_DRV48_1P8
Model_648 I/O,1.8V,SR000_DRV48_1P8
Model_649 I/O,1.8V,SR011_DRV40_1P8
Model_650 I/O,1.8V,SR010_DRV40_1P8
Model_651 I/O,1.8V,SR101_DRV40_1P8
Model_652 I/O,1.8V,SR100_DRV40_1P8
Model_653 I/O,1.8V,SR110_DRV40_1P8
Model_654 I/O,1.8V,SR111_DRV40_1P8
Model_655 I/O,1.8V,SR001_DRV40_1P8
Model_656 I/O,1.8V,SR000_DRV40_1P8
Model_657 I/O,1.8V,SR011_DRV34_1P8
Model_658 I/O,1.8V,SR010_DRV34_1P8
Model_659 I/O,1.8V,SR101_DRV34_1P8
Model_660 I/O,1.8V,SR100_DRV34_1P8
Model_661 I/O,1.8V,SR110_DRV34_1P8
Model_662 I/O,1.8V,SR111_DRV34_1P8
Model_663 I/O,1.8V,SR001_DRV34_1P8
Model_664 I/O,1.8V,SR000_DRV34_1P8
Model_674 I/O,1.5V,SR011_DRV40_1P5
Model_675 I/O,1.5V,SR010_DRV40_1P5
Model_676 I/O,1.5V,SR101_DRV40_1P5
Model_677 I/O,1.5V,SR100_DRV40_1P5
Model_678 I/O,1.5V,SR110_DRV40_1P5
Model_679 I/O,1.5V,SR111_DRV40_1P5
Model_680 I/O,1.5V,SR001_DRV40_1P5
Model_681 I/O,1.5V,SR000_DRV40_1P5
Model_682 I/O,1.5V,SR011_DRV34_1P5
Model_683 I/O,1.5V,SR010_DRV34_1P5
Model_684 I/O,1.5V,SR101_DRV34_1P5
Model_685 I/O,1.5V,SR100_DRV34_1P5
Model_686 I/O,1.5V,SR110_DRV34_1P5
Model_687 I/O,1.5V,SR111_DRV34_1P5
Model_688 I/O,1.5V,SR001_DRV34_1P5
Model_689 I/O,1.5V,SR000_DRV34_1P5
Model_690 I/O,1.5V,SR011_DRV48_1P5
Model_691 I/O,1.5V,SR010_DRV48_1P5
Model_692 I/O,1.5V,SR101_DRV48_1P5
Model_693 I/O,1.5V,SR100_DRV48_1P5
Model_694 I/O,1.5V,SR110_DRV48_1P5
Model_695 I/O,1.5V,SR111_DRV48_1P5
Model_696 I/O,1.5V,SR001_DRV48_1P5
Model_697 I/O,1.5V,SR000_DRV48_1P5
Model_698 I/O,1.35V,SR011_DRV40_1P35
Model_699 I/O,1.35V,SR010_DRV40_1P35
Model_700 I/O,1.35V,SR101_DRV40_1P35
Model_701 I/O,1.35V,SR100_DRV40_1P35
Model_702 I/O,1.35V,SR110_DRV40_1P35
Model_703 I/O,1.35V,SR111_DRV40_1P35
Model_704 I/O,1.35V,SR001_DRV40_1P35
Model_705 I/O,1.35V,SR000_DRV40_1P35
Model_706 I/O,1.35V,SR011_DRV34_1P35
Model_707 I/O,1.35V,SR010_DRV34_1P35
Model_708 I/O,1.35V,SR101_DRV34_1P35
Model_709 I/O,1.35V,SR100_DRV34_1P35
Model_710 I/O,1.35V,SR110_DRV34_1P35
Model_711 I/O,1.35V,SR111_DRV34_1P35
Model_712 I/O,1.35V,SR001_DRV34_1P35
Model_713 I/O,1.35V,SR000_DRV34_1P35
Model_714 I/O,1.35V,SR011_DRV48_1P35
Model_715 I/O,1.35V,SR010_DRV48_1P35
Model_716 I/O,1.35V,SR101_DRV48_1P35
Model_717 I/O,1.35V,SR100_DRV48_1P35
Model_718 I/O,1.35V,SR110_DRV48_1P35
Model_719 I/O,1.35V,SR111_DRV48_1P35
Model_720 I/O,1.35V,SR001_DRV48_1P35
Model_721 I/O,1.35V,SR000_DRV48_1P35
|   Usage I/O#1.8/3###SDIO1833PB_H.PAD
|   Base model SDIO1833PB_H
[Model Selector] Selector_8
Model_178 I/O,3V,50OHMS_3
Model_179 I/O,3V,66OHMS_3
Model_180 I/O,3V,33OHMS_3
Model_181 I/O,3V,100OHMS_3
Model_182 I/O,1.8V,50OHMS_1P8
Model_183 I/O,1.8V,66OHMS_1P8
Model_184 I/O,1.8V,33OHMS_1P8
Model_185 I/O,1.8V,100OHMS_1P8
|   Usage I/O#1.35/1.5/1.8###DDR_SEIOPB_H.PAD
|   Base model DDR_SEIOPB_H
[Model Selector] Selector_9
Model_100 I/O,1.8V,SR111_DRV40_1P8
Model_101 I/O,1.8V,SR001_DRV40_1P8
Model_102 I/O,1.8V,SR000_DRV40_1P8
Model_103 I/O,1.8V,SR011_DRV34_1P8
Model_104 I/O,1.8V,SR010_DRV34_1P8
Model_105 I/O,1.8V,SR101_DRV34_1P8
Model_106 I/O,1.8V,SR100_DRV34_1P8
Model_107 I/O,1.8V,SR110_DRV34_1P8
Model_108 I/O,1.8V,SR111_DRV34_1P8
Model_109 I/O,1.8V,SR001_DRV34_1P8
Model_110 I/O,1.8V,SR000_DRV34_1P8
Model_111 INPUT,1.5V,DDR3_ODT_80_1P5
Model_112 INPUT,1.5V,DDR3_ODT_60_1P5
Model_113 INPUT,1.5V,DDR3_ODT_120_1P5
Model_114 INPUT,1.35V,DDR3L_ODT_80_1P35
Model_115 INPUT,1.35V,DDR3L_ODT_60_1P35
Model_116 INPUT,1.35V,DDR3L_ODT_120_1P35
Model_117 INPUT,1.8V,DDR2_ODT_120_1P8
Model_118 INPUT,1.8V,DDR2_ODT_80_1P8
Model_119 INPUT,1.8V,DDR2_ODT_60_1P8
Model_120 I/O,1.5V,SR011_DRV40_1P5
Model_121 I/O,1.5V,SR010_DRV40_1P5
Model_122 I/O,1.5V,SR101_DRV40_1P5
Model_123 I/O,1.5V,SR100_DRV40_1P5
Model_124 I/O,1.5V,SR110_DRV40_1P5
Model_125 I/O,1.5V,SR111_DRV40_1P5
Model_126 I/O,1.5V,SR001_DRV40_1P5
Model_127 I/O,1.5V,SR000_DRV40_1P5
Model_128 I/O,1.5V,SR011_DRV34_1P5
Model_129 I/O,1.5V,SR010_DRV34_1P5
Model_130 I/O,1.5V,SR101_DRV34_1P5
Model_131 I/O,1.5V,SR100_DRV34_1P5
Model_132 I/O,1.5V,SR110_DRV34_1P5
Model_133 I/O,1.5V,SR111_DRV34_1P5
Model_134 I/O,1.5V,SR001_DRV34_1P5
Model_135 I/O,1.5V,SR000_DRV34_1P5
Model_136 I/O,1.5V,SR011_DRV48_1P5
Model_137 I/O,1.5V,SR010_DRV48_1P5
Model_138 I/O,1.5V,SR101_DRV48_1P5
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| Models and submodels in the file (413): Model_1 (Input), Model_2 (Input), Model_3 (3-state), Model_4 (3-state), Model_5 (Input), Model_6 (Input), Model_87 (I/O), Model_88 (I/O), Model_89 (I/O), Model_90 (I/O), Model_91 (I/O), Model_92 (I/O), Model_93 (I/O), Model_94 (I/O), Model_95 (I/O), Model_96 (I/O), Model_97 (I/O), Model_98 (I/O), Model_99 (I/O), Model_100 (I/O), Model_101 (I/O), Model_102 (I/O), Model_103 (I/O), Model_104 (I/O), Model_105 (I/O), Model_106 (I/O), Model_107 (I/O), Model_108 (I/O), Model_109 (I/O), Model_110 (I/O), Model_111 (Input), Model_112 (Input), Model_113 (Input), Model_114 (Input), Model_115 (Input), Model_116 (Input), Model_117 (Input), Model_118 (Input), Model_119 (Input), Model_120 (I/O), Model_121 (I/O), Model_122 (I/O), Model_123 (I/O), Model_124 (I/O), Model_125 (I/O), Model_126 (I/O), Model_127 (I/O), Model_128 (I/O), Model_129 (I/O), Model_130 (I/O), Model_131 (I/O), Model_132 (I/O), Model_133 (I/O), Model_134 (I/O), Model_135 (I/O), Model_136 (I/O), Model_137 (I/O), Model_138 (I/O), Model_139 (I/O), Model_140 (I/O), Model_141 (I/O), Model_142 (I/O), Model_143 (I/O), Model_144 (I/O), Model_145 (I/O), Model_146 (I/O), Model_147 (I/O), Model_148 (I/O), Model_149 (I/O), Model_150 (I/O), Model_151 (I/O), Model_152 (I/O), Model_153 (I/O), Model_154 (I/O), Model_155 (I/O), Model_156 (I/O), Model_157 (I/O), Model_158 (I/O), Model_159 (I/O), Model_160 (I/O)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
